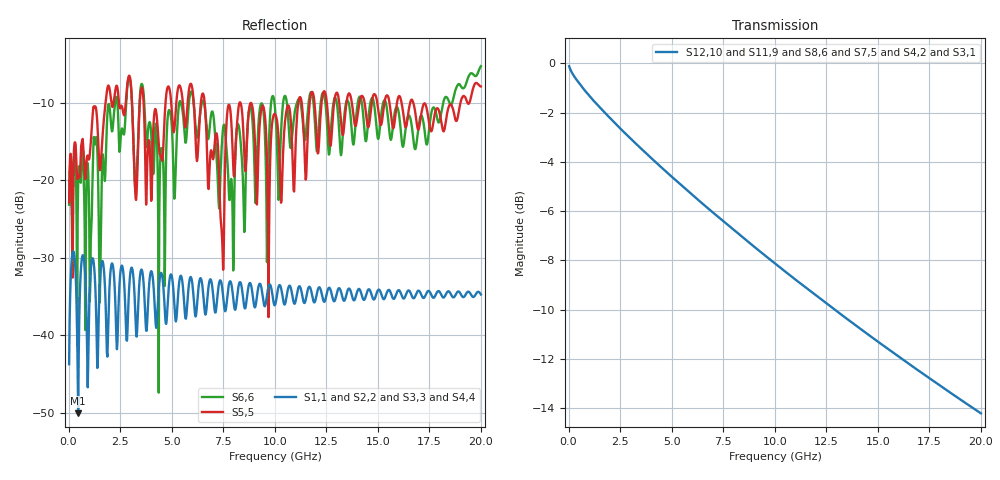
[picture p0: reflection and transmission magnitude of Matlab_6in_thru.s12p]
! Generated by program util_makeSnpFromS4p on 02-16-2011 11:10:43
! Thru channel ports
!  1-----xxxxxxxxxxxxxxxxxx----- 3
!  xxxxxxxxxxxxxxxxxx
!  (Input) xxxxxxxxxxxxxxxxxx  (Output)
!  xxxxxxxxxxxxxxxxxx
!  2-----xxxxxxxxxxxxxxxxxx----- 4
! Crosstalk 1 input ports are {(5),(6)}.
! Crosstalk 2 input ports are {(9),(10)}.
! Crosstalk n input ports are {(4n+1),(4n+2)}.
! All crosstalk output ports are {(3),(4)}.
# Hz S DB R 50
! Freq  S11  S12  S13  S14
!  S15  S16  S17  S18
!  S19  S110  S111  S112
!  S21  S22  S23  S24
!  S25  S26  S27  S28
!  S29  S210  S211  S212
!  S31  S32  S33  S34
!  S35  S36  S37  S38
!  S39  S310  S311  S312
!  S41  S42  S43  S44
!  S45  S46  S47  S48
!  S49  S410  S411  S412
!  S51  S52  S53  S54
!  S55  S56  S57  S58
!  S59  S510  S511  S512
!  S61  S62  S63  S64
!  S65  S66  S67  S68
!  S69  S610  S611  S612
!  S71  S72  S73  S74
!  S75  S76  S77  S78
!  S79  S710  S711  S712
!  S81  S82  S83  S84
!  S85  S86  S87  S88
!  S89  S810  S811  S812
!  S91  S92  S93  S94
!  S95  S96  S97  S98
!  S99  S910  S911  S912
!  S101  S102  S103  S104
!  S105  S106  S107  S108
!  S109  S1010  S1011  S1012
!  S111  S112  S113  S114
!  S115  S116  S117  S118
!  S119  S1110  S1111  S1112
!  S121  S122  S123  S124
!  S125  S126  S127  S128
!  S129  S1210  S1211  S1212
!  (dB)  (deg)  (dB)  (deg)  (dB)  (deg)  (dB)  (deg)
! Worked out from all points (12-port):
!   819 points, 24.41 MHz to 20 GHz, reference 50 ohm
!   strongest paths, dB at 24.41 MHz, 5.005 GHz, 10.01 GHz, 15.02 GHz, 20 GHz:
!     S12,10: -0.1, -4.6, -8.1, -11.3, -14.2
!     S11,9: -0.1, -4.6, -8.1, -11.3, -14.2
!     S8,6: -0.1, -4.6, -8.1, -11.3, -14.2
!     S7,5: -0.1, -4.6, -8.1, -11.3, -14.2
!     S4,2: -0.1, -4.6, -8.1, -11.3, -14.2
!     S3,1: -0.1, -4.6, -8.1, -11.3, -14.2
!   lowest |S11| = -50.0 dB at 463.9 MHz (marker M1), VSWR 1.01, Z = 49.7 - j0.09 ohm
!   |S11| at or under -10 dB: start of sweep to end of sweep
